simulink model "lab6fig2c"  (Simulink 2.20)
settings: Solver=ode45  StartTime=0.0  StopTime=10.0  MaxStep=0.01  RelTol=1e-3  AbsTol=1e-6
libraries: simulink x2

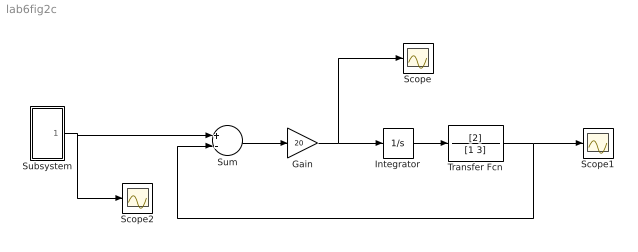
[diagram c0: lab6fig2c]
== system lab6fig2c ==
  Gain : Gain  Gain=20
  Integrator : Integrator  ExternalReset=none  InitialConditionSource=internal  InitialCondition=0  LimitOutput=off  UpperSaturationLimit=inf  LowerSaturationLimit=-inf  ShowSaturationPort=off  ShowStatePort=off  AbsoluteTolerance=auto
  Scope : Scope
  Scope1 : Scope
  Scope2 : Scope
  Subsystem : Subsystem
  Sum : Sum  Inputs=+-
  Transfer Fcn : TransferFcn  Numerator=[2]  Denominator=[1 3]
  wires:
  Sum/1 -> Gain/1
  Integrator/1 -> Transfer Fcn/1
  Gain/1 -> Integrator/1, Scope/1
  Transfer Fcn/1 -> Scope1/1, Sum/2
  Subsystem/1(Out1) -> Sum/1, Scope2/1

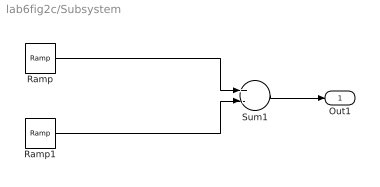
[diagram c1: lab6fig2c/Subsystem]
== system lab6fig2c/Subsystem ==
  Ramp : simulink/Sources/Ramp  slope=1  start=0  X0=0
  Ramp1 : simulink/Sources/Ramp  slope=1  start=1  X0=0
  Sum1 : Sum  Inputs=+-
  Out1 : Outport  Port=1
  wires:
  Sum1/1 -> Out1/1
  Ramp/1 -> Sum1/1
  Ramp1/1 -> Sum1/2
